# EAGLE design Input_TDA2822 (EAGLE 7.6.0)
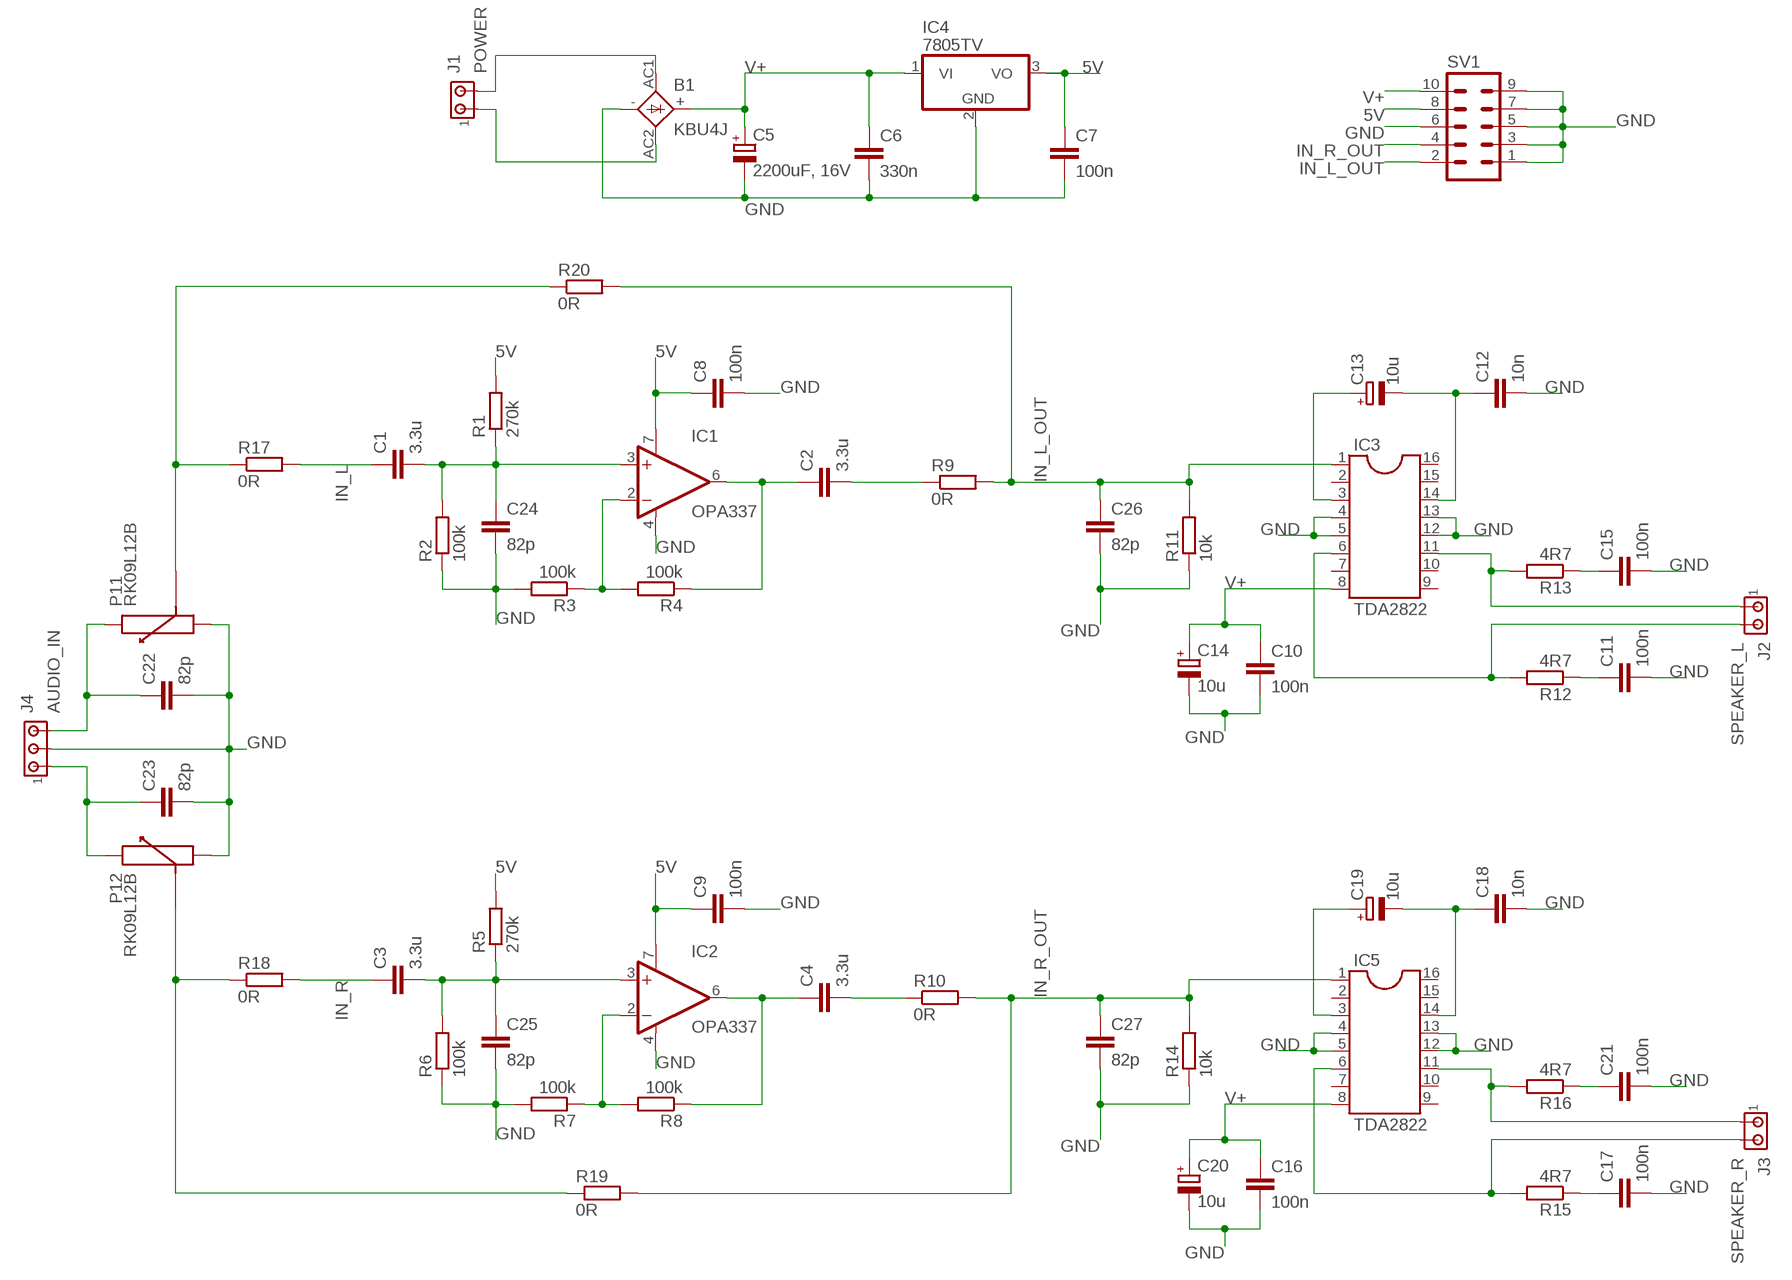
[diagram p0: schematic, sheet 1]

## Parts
B1  KBU4J  KBU  [KBU]
C1  3.3u  C-EU050-055X075  [C050-055X075]
C2  3.3u  C-EU050-055X075  [C050-055X075]
C3  3.3u  C-EU050-055X075  [C050-055X075]
C4  3.3u  C-EU050-055X075  [C050-055X075]
C5  2200uF, 16V  CPOL-EUE5-13  [E5-13]
C6  330n  C-EU050-035X075  [C050-035X075]
C7  100n  C-EU050-025X075  [C050-025X075]
C8  100n  C-EU050-025X075  [C050-025X075]
C9  100n  C-EU050-025X075  [C050-025X075]
C10  100n  C-EU050-025X075  [C050-025X075]
C11  100n  C-EU050-025X075  [C050-025X075]
C12  10n  C-EU025-025X050  [C025-025X050]
C13  10u  CPOL-EUE2-5  [E2-5]
C14  10u  CPOL-EUE2-5  [E2-5]
C15  100n  C-EU050-025X075  [C050-025X075]
C16  100n  C-EU050-025X075  [C050-025X075]
C17  100n  C-EU050-025X075  [C050-025X075]
C18  10n  C-EU025-025X050  [C025-025X050]
C19  10u  CPOL-EUE2-5  [E2-5]
C20  10u  CPOL-EUE2-5  [E2-5]
C21  100n  C-EU050-025X075  [C050-025X075]
C22  82p  C-EU025-024X044  [C025-024X044]
C23  82p  C-EU025-024X044  [C025-024X044]
C24  82p  C-EU025-024X044  [C025-024X044]
C25  82p  C-EU025-024X044  [C025-024X044]
C26  82p  C-EU025-024X044  [C025-024X044]
C27  82p  C-EU025-024X044  [C025-024X044]
IC1  OPA337  OPA336P  [DIL08]
IC2  OPA337  OPA336P  [DIL08]
IC3  TDA2822  DIL16S  [SOCKET-16]
IC4  7805TV  [TO220V]
IC5  TDA2822  DIL16S  [SOCKET-16]
J1  POWER  350428-1  [350428-1]
J2  SPEAKER_L  350428-1  [350428-1]
J3  SPEAKER_R  350428-1  [350428-1]
J4  AUDIO_IN  350429-1  [350429-1]
P1  RK09L12B  [ALPS-RK09L12B0]
R1  270k  R-EU_0309/V  [0309V]
R2  100k  R-EU_0309/V  [0309V]
R3  100k  R-EU_0309/V  [0309V]
R4  100k  R-EU_0309/V  [0309V]
R5  270k  R-EU_0309/V  [0309V]
R6  100k  R-EU_0309/V  [0309V]
R7  100k  R-EU_0309/V  [0309V]
R8  100k  R-EU_0309/V  [0309V]
R9  0R  R-EU_R0603  [R0603]
R10  0R  R-EU_R0603  [R0603]
R11  10k  R-EU_0309/V  [0309V]
R12  4R7  R-EU_0309/V  [0309V]
R13  4R7  R-EU_0309/V  [0309V]
R14  10k  R-EU_0309/V  [0309V]
R15  4R7  R-EU_0309/V  [0309V]
R16  4R7  R-EU_0309/V  [0309V]
R17  0R  R-EU_R0603  [R0603]
R18  0R  R-EU_R0603  [R0603]
R19  0R  R-EU_R0603  [R0603]
R20  0R  R-EU_R0603  [R0603]
SV1  ML10  [ML10]

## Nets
5V: C7.1 C8.1 C9.1 IC1.7(V+) IC2.7(V+) IC4.3(VO) R1.2 R5.2 SV1.8
GND: B1.- C5.- C6.2 C7.2 C8.2 C9.2 C10.2 C11.2 C12.2 C14.- C15.2 C16.2 C17.2 C18.2 C20.- C21.2 C22.2 C23.2 C24.2 C25.2 C26.2 C27.2 IC1.4(V-) IC2.4(V-) IC3.4 IC3.5 IC3.12 IC3.13 IC4.2(GND) IC5.4 IC5.5 IC5.12 IC5.13 J4.2 P1.GND1(1:GND$1) P1.GND2(2:GND$1) R2.1 R3.2 R6.1 R7.2 R11.1 R14.1 SV1.1 SV1.3 SV1.5 SV1.6 SV1.7 SV1.9
IN_L: C1.1 R17.2
IN_L_OUT: C26.1 IC3.1 R9.2 R11.2 R20.2 SV1.2
IN_R: C3.1 R18.2
IN_R_OUT: C27.1 IC5.1 R10.2 R14.2 R19.2 SV1.4
N$1: C1.2 C24.1 IC1.3(+IN) R1.1 R2.2
N$2: C3.2 C25.1 IC2.3(+IN) R5.1 R6.2
N$3: IC1.2(-IN) R3.1 R4.2
N$4: IC2.2(-IN) R7.1 R8.2
N$5: C2.1 IC1.6(OUT) R4.1
N$6: C4.1 IC2.6(OUT) R8.1
N$7: B1.AC1 J1.2
N$8: B1.AC2 J1.1
N$10: IC3.6 J2.2 R12.2
N$12: C2.2 R9.1
N$14: C19.+ IC5.3
N$15: C13.+ IC3.3
N$16: C12.1 C13.- IC3.14
N$17: C11.1 R12.1
N$18: C18.1 C19.- IC5.14
N$19: IC5.6 J3.2 R15.2
N$20: C17.1 R15.1
N$21: IC3.11 J2.1 R13.2
N$22: C15.1 R13.1
N$23: IC5.11 J3.1 R16.2
N$24: C21.1 R16.1
N$25: C22.1 J4.3 P1.IN1(1:IN$1)
N$27: C23.1 J4.1 P1.IN2(2:IN$1)
N$28: P1.OUT2(2:OUT$1) R18.1 R19.1
N$29: P1.OUT1(1:OUT$1) R17.1 R20.1
N$30: C4.2 R10.1
V+: B1.+ C5.+ C6.1 C10.1 C14.+ C16.1 C20.+ IC3.8 IC4.1(VI) IC5.8 SV1.10
Unconnected: IC3.2 IC3.7 IC3.9 IC3.10 IC3.15 IC3.16 IC5.2 IC5.7 IC5.9 IC5.10 IC5.15 IC5.16

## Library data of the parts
B1 = rectifier:KBU: DIOTEC RECTIFIER
C1-C4 C6-C12 C15-C18 C21-C27 = rcl:C-EU: CAPACITOR, European symbol
C5 C13 C14 C19 C20 = rcl:CPOL-EU: POLARIZED CAPACITOR, European symbol
IC1 IC2 = burr-brown:OPA336: CMOS Operational Amplifiers Single-Supply, MicroPower, MicroAmplifier(TM) Series; OC_FARNELL: unknown; OC_NEWARK: unknown
IC3 IC5 = ic-package:DIL16: Dual In Line / Socket
IC4 = linear:78*: Positive VOLTAGE REGULATOR Source: http://cache.national.com/ds/LM/LM78L05.pdf http://www.fairchildsemi.com/ds/LM/LM7805.pdf
J1-J3 = con-amp:350428-1: Universal MATE-N-LOK .250" Centerline, 600 V, 19 - 36 A max
J4 = con-amp:350429-1: Universal MATE-N-LOK .250" Centerline, 600 V, 19 - 36 A max Source: http://catalog.tycoelectronics.com/ .. ENG_CD_350429_Y.pdf
P1 = my:RK09L12B
R1-R20 = rcl:R-EU_: RESISTOR, European symbol
SV1 = con-ml:ML10: HARTING; OC_FARNELL: unknown; OC_NEWARK: unknown

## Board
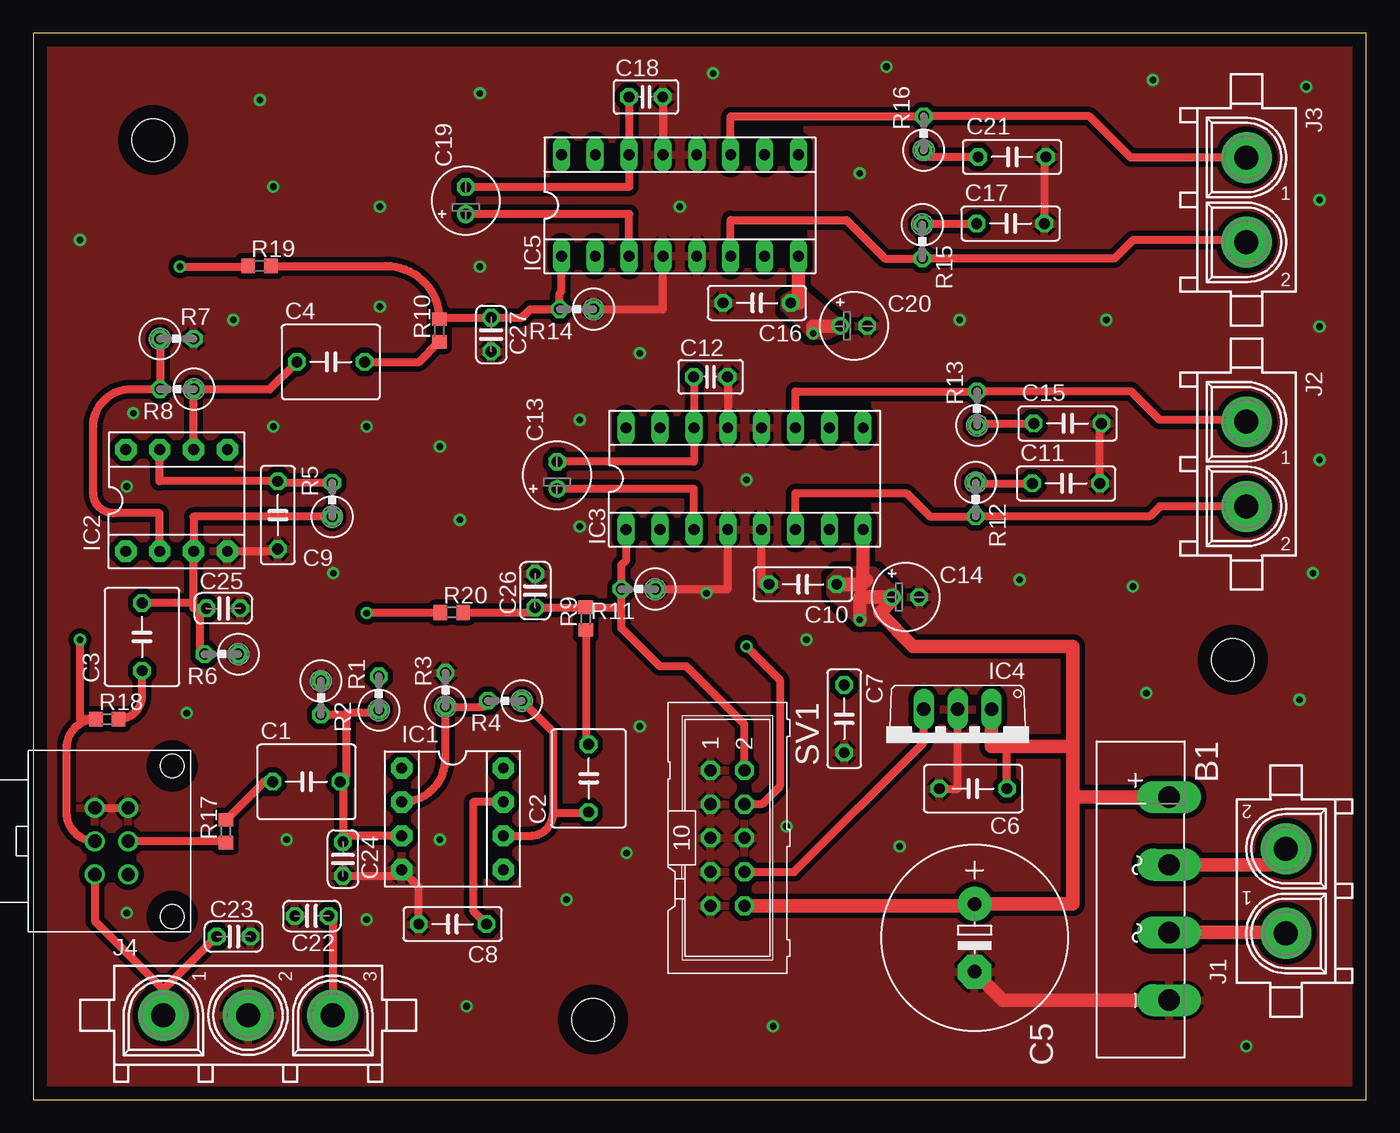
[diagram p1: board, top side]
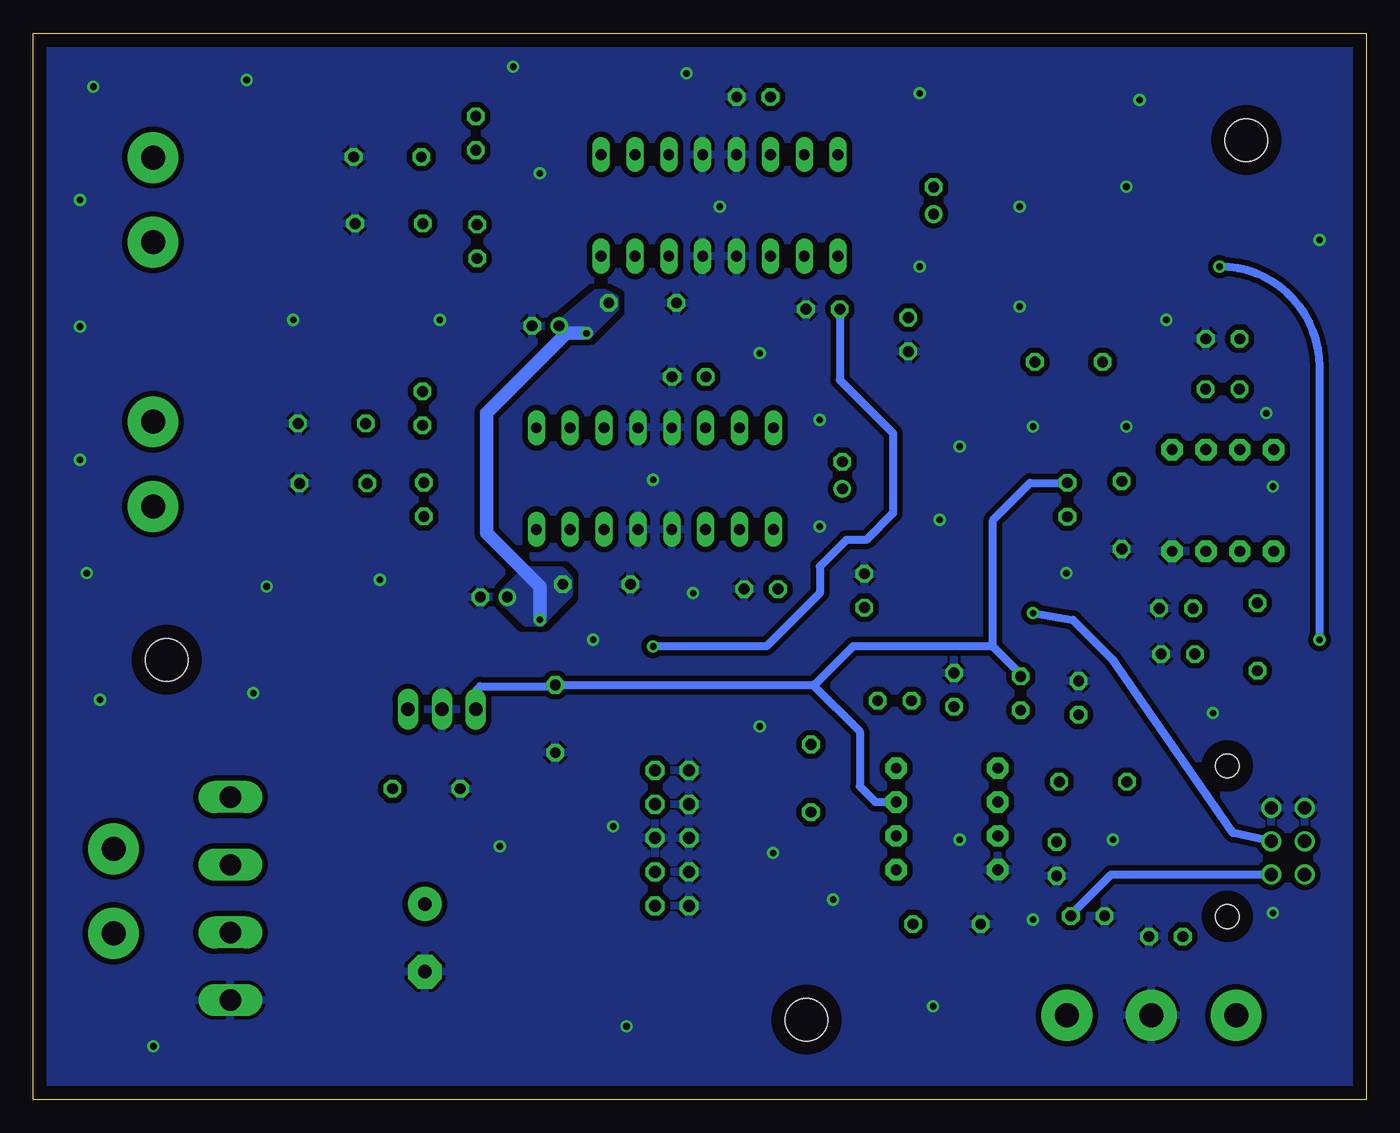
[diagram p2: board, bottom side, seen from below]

Size 100 x 80 mm. Coordinates in mm from the lower left corner, seen from the top.
Outline: 0,0 100,0 100,80 0,80 0,0
Copper layers (1*16): Top 0.035mm / dielectric 1.5mm / Bottom 0.035mm
Design rules "default": minimum track width 10mil, minimum drill 24mil, track to track 8mil, track to pad 8mil, pad to pad 8mil, via to via 8mil, smd to smd 8mil, copper to edge 40mil, drill to drill 8mil, minimum pad ring 10mil, minimum via ring 8mil, stop-mask expansion 4mil, vias tented up to drill 0mil, thermal gap 10mil
Holes 3.2 mm at 9,72 90,33 42,6

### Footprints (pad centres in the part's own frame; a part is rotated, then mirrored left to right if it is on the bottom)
KBU = drill 1.6 long: + -7.62,2.54; - 7.62,2.54; AC1 -2.54,2.54; AC2 2.54,2.54
C050-055X075 = drill 0.813 octagon: 1 -2.54,0; 2 2.54,0
E5-13 = drill 1.016 pad 2.54: + -2.54,0 | drill 1.016 pad 2.54 octagon: - 2.54,0
C050-035X075 = drill 0.813 octagon: 1 -2.54,0; 2 2.54,0
C050-025X075 = drill 0.813 octagon: 1 -2.54,0; 2 2.54,0
C025-025X050 = drill 0.813 octagon: 1 -1.27,0; 2 1.27,0
E2-5 = drill 0.813 pad 1.27: + -1.016,0 | drill 0.813 pad 1.27 octagon: - 1.016,0
C025-024X044 = drill 0.813 octagon: 1 -1.27,0; 2 1.27,0
DIL08 = drill 0.813 pad 1.6 octagon: 1 -3.81,-3.81; 2 -1.27,-3.81; 3 1.27,-3.81; 4 3.81,-3.81; 5 3.81,3.81; 6 1.27,3.81; 7 -1.27,3.81; 8 -3.81,3.81
SOCKET-16 = drill 0.813 long: 1 -8.89,-3.81; 2 -6.35,-3.81; 3 -3.81,-3.81; 4 -1.27,-3.81; 5 1.27,-3.81; 6 3.81,-3.81; 7 6.35,-3.81; 8 8.89,-3.81; 9 8.89,3.81; 10 6.35,3.81; 11 3.81,3.81; 12 1.27,3.81; 13 -1.27,3.81; 14 -3.81,3.81; 15 -6.35,3.81; 16 -8.89,3.81
TO220V = drill 1.016 long: 1 -2.54,-2.54; 2 0,-2.54; 3 2.54,-2.54
350428-1 = drill 1.8 pad 3.81: 1 -3.175,0; 2 3.175,0
350429-1 = drill 1.8 pad 3.81: 1 -6.35,0; 2 0,0; 3 6.35,0
ALPS-RK09L12B0 = drill 1: GND1 3.3,-2.5; GND2 5.8,-2.5; IN1 3.3,2.5; IN2 5.8,2.5; OUT1 3.3,0; OUT2 5.8,0 | hole 1.8: 0,-5.65; 0,5.65
0309V = drill 0.813 octagon: 1 -1.27,0; 2 1.27,0
R0603 = smd 1 x 1.1: 1 -0.85,0; 2 0.85,0
ML10 = drill 0.914 octagon: 1 -5.08,-1.27; 2 -5.08,1.27; 3 -2.54,-1.27; 4 -2.54,1.27; 5 0,-1.27; 6 0,1.27; 7 2.54,-1.27; 8 2.54,1.27; 9 5.08,-1.27; 10 5.08,1.27

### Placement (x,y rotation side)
B1  82.68,15.07 270 top
C1  20.49,23.84 0 top
C2  41.66,24.1 90 top
C3  8.16,34.71 90 top
C4  22.32,55.34 0 top
C5  70.62,12.13 270 top
C6  70.51,23.32 180 top
C7  60.84,28.57 270 top
C8  31.46,13.16 180 top
C9  18.34,43.85 270 top
C10  57.74,38.66 180 top
C11  77.49,46.23 0 top
C12  50.81,54.23 0 top
C13  39.3,46.84 90 top
C14  65.45,37.7 0 top
C15  77.6,50.73 0 top
C16  54.29,59.77 180 top
C17  73.32,65.73 0 top
C18  45.96,75.23 0 top
C19  32.45,67.45 90 top
C20  61.56,58.05 0 top
C21  73.43,70.73 0 top
C22  20.89,13.77 180 top
C23  15.03,12.23 0 top
C24  23.23,18.05 270 top
C25  14.26,36.85 0 top
C26  37.65,38.18 90 top
C27  34.35,57.4 270 top
IC1  31.45,21.05 270 top
IC2  10.75,44.95 0 top
IC3  53.37,46.59 0 top
IC4  69.35,26.74 180 top
IC5  48.51,67.09 0 top
J1  93.98,15.64 90 top
J2  91.02,47.68 270 top
J3  91.02,67.5 270 top
J4  16.11,6.32 0 top
P1  10.42,19.38 180 top
R1  25.92,30.48 90 top
R2  21.58,30.14 270 top
R3  30.92,30.74 90 top
R4  35.38,29.92 180 top
R5  22.42,45 90 top
R6  14.12,33.42 180 top
R7  10.76,57.08 0 top
R8  10.78,53.3 180 top
R9  41.45,36.08 90 top
R10  30.45,57.71 90 top
R11  45.4,38.3 180 top
R12  70.7,45.02 270 top
R13  70.8,51.86 90 top
R14  40.76,59.3 180 top
R15  66.7,64.38 270 top
R16  66.8,72.5 90 top
R17  14.45,20.13 90 top
R18  5.55,28.55 0 top
R19  16.97,62.55 0 top
R20  31.39,36.55 0 top
SV1  52.08,19.62 270 top

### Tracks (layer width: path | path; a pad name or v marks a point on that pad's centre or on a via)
5V
  Top 0.61: IC2.7 9.48,46.39 C9.1 18.34,46.27 R5.2 | IC1.7 33,22.32 33,14.16 C8.1 | SV1.8 57.08,17.08 66.81,26.81 IC4.3
  Bottom 0.61: IC4.3 66.81,30.69 66.5,31 60.45,31 C7.1 41.5,31.11 | 41.5,31.11 41.39,31.11 38.5,34 28,34 | IC1.7 36.82,22.32 38,23.5 38,27.61 41.5,31.11 | 28,34 28,43.5 25.23,46.27 R5.2 | R1.2 26.25,32.25 28,34
GND  (via drill 0.5)
  Top 0.61: J4.2 16.3,6.51 | P1.GND2 P1.GND1 | IC2.4 18.34,41.14 C9.2 | C24.2 27.18,16.78 IC1.4 28.92,15.96 C8.2 | C10.2 54.64,38.66 IC3.5 | C11.2 80.03,50.73 C15.2 | C18.2 IC5.13 | C12.2 52.1,54.23 IC3.13 | R11.1 52.1,38.3 IC3.4 | R14.1 47.24,59.3 IC5.4 | C21.2 75.86,70.62 C17.2 | C6.2 69.35,23.32 IC4.2
  Top 1.016: B1.- 72.76,7.45 C5.-
  other vias: 17,75 30.5,49 45.5,56 48.5,67 51,77 62,69.5 84,76.5 80.5,58.5 69.5,58.5 82.5,38.5 74,39 83.5,30.5 50.5,38 45.5,28 40,15 22.5,39.5 11.5,29 3.5,64.5 7,46 18,50.5 26,59.5 26,67 7.5,51.5 33.5,62.5 41,51 32,43.5 41,43 44.5,18.5 30.5,19.5 25,13.5 19,19.5 7,14 32.5,7 55.5,5.5 91,4 95,30 65,19 58,34.5 56.5,20.5 64,77.5 96.5,58 95.5,76 96,39.5 96.5,48 96.5,67.5 33.5,75.5 18,68.5 25,50.5 15,58.5 53.5,46.5
  pour Top (isolate 0.406, rank 2): 0.5,79.5 0.5,0.5 99.5,0.5 99.5,79.5
  pour Bottom (isolate 0.406, rank 2): 0.5,79.5 0.5,0.5 99.5,0.5 99.5,79.5
IN_L
  Top 0.61: R17.2 17.31,23.84 C1.1
IN_L_OUT
  Top 0.61: R11.2 44.13,40.13 44.5,40.5 44.5,42.76 IC3.1 | R20.2 37.29,36.55 C26.1 41.43,36.91 R9.2 44.13,36.93 R11.2 | SV1.2 53.35,28.15 49,32.5 47,32.5 44.13,35.37 R11.2
IN_R
  Top 0.61: R18.2 arc90 8.16,30.31 C3.1
IN_R_OUT  (via drill 0.5)
  Top 0.61: IC5.1 39.62,60.62 39.49,60.49 R14.2 37.3,59.3 36.67,58.67 C27.1 30.56,58.67 R10.2 arc90 26.46,62.55 R19.2 | SV1.4 54.66,22.16 56,23.5 56,31.5 v53.5,34
  Bottom 0.61: R14.2 39.49,53.99 35.5,50 35.5,44 37.5,42 39,42 41,40 41,38 45,34 v53.5,34
N$1
  Top 0.61: IC1.3 23.69,19.78 C24.1 23.23,23.64 C1.2 23.5,24.31 23.5,29 | 23.5,29 23.37,28.87 R2.2 | R1.1 25.71,29 23.5,29
N$2
  Top 0.61: IC2.3 arc90 12,41.12 12,39 | 12.02,37.25 C3.2 | 12.02,37.25 IC2.3 | C25.1 12.5,36.85 | 12.5,36.85 12.02,36.85 12.02,37.25 | R6.2 12.5,33.42 12.5,36.85 | R5.1 12.02,43.73 IC2.3
N$3
  Top 0.61: IC1.2 arc90 30.92,25.6 R3.1 33.66,29.47 arc90 R4.2
N$4
  Top 0.61: IC2.2 9.48,44 6,44 arc-90 4.5,45.5 4.5,50.5 arc-90 7.3,53.3 R8.2 9.51,57.06 arc90 R7.1
N$5
  Top 0.61: IC1.6 37.28,19.78 arc90 39,21.5 | 39,21.5 41.6,21.5 arc90 C2.1 | R4.1 39,27.57 39,21.5
N$6
  Top 0.61: C4.1 17.74,53.3 R8.1 12.02,53.27 IC2.6
N$7
  Top 1.016: J1.2 92.78,17.61 B1.AC1
N$8
  Top 1.016: J1.1 93.92,12.53 B1.AC2
N$10
  Top 0.61: IC3.6 57.18,45.5 65.5,45.5 67.25,43.75 R12.2 83.75,43.75 84.5,44.5 J2.2
N$12
  Top 0.61: R9.1 41.45,26.85 C2.2
N$14
  Top 0.61: IC5.3 44.7,66.43 C19.+
N$15
  Top 0.61: IC3.3 49.56,45.82 C13.+
N$16
  Top 0.61: C12.1 49.56,54.23 IC3.14 49.56,47.86 C13.-
N$17
  Top 0.61: R12.1 70.7,46.23 C11.1
N$18
  Top 0.61: C18.1 IC5.14 44.7,68.47 C19.-
N$19
  Top 0.61: J3.2 90.84,64.5 82.5,64.5 81.11,63.11 R15.2 63.89,63.11 61,66 52.32,66 IC5.6
N$20
  Top 0.61: R15.1 66.78,65.73 C17.1
N$21
  Top 0.61: J2.1 90.88,51 84.5,51 82.37,53.13 R13.2 57.18,53.13 IC3.11
N$22
  Top 0.61: R13.1 70.8,50.73 C15.1
N$23
  Top 0.61: IC5.11 52.32,73.77 R16.2 79.23,73.77 82.33,70.67 J3.1
N$24
  Top 0.61: R16.1 67.3,70.73 C21.1
N$25
  Top 0.61: J4.3 22.5,6.36 22.5,13.43 C22.1
  Bottom 0.61: C22.1 22.16,13.84 19.12,16.88 P1.IN1
N$27
  Top 0.61: 9.76,8.26 J4.1 | P1.IN2 4.62,13.4 9.76,8.26 | 9.76,8.26 9.79,8.26 C23.1
N$28  (via drill 0.5)
  Top 0.61: P1.OUT2 arc-90 2.5,21.5 2.5,26.35 arc-90 R18.1 3.5,28.55 v3.5,34.5 | v11,62.5 16.07,62.5 arc90 R19.1
  Bottom 0.61: v3.5,34.5 3.5,55 arc-90 v11,62.5
N$29  (via drill 0.5)
  Top 0.61: R20.1 30.49,36.5 v25,36.5 | R17.1 14.35,19.38 P1.OUT1
  Bottom 0.61: v25,36.5 22,36 19,33 10,20 P1.OUT1
N$30
  Top 0.61: C4.2 28.93,55.34 R10.1
V+  (via drill 0.5)
  Top 0.61: C6.1 73.05,26.5 74.5,26.5
  Top 1.016: B1.+ 78,22.69 | 78,22.69 78,26.5 | 78,26.5 74.5,26.5 71.89,26.5 IC4.1 | 78,22.69 78,14.67 C5.+ 70.62,14.54 SV1.10 | C20.+ 58.5,58.05 v58.5,57.5 | v62,36 62,37.7 C14.+ 64.43,37.43 63.5,36.5 66,34 78,34 78,26.5 | IC3.8 62.26,39.24 62.5,39 62.16,38.66 C10.1 | IC5.8 57.4,59.77 C16.1
  Bottom 1.016: v62,36 62,38.5 66,42.5 66,51.5 60,57.5 v58.5,57.5
  pour Top (isolate 0.406, no thermals): 58.5,57.5 56.5,59.5 56.5,60 57.5,60.5 60.5,58 59.5,57.5
  pour Bottom (isolate 0.406, no thermals): 58.5,57.5 56.5,59.5 56.5,60 57.5,60.5 60.5,58 59.5,57.5
  pour Bottom (isolate 0.406, no thermals): 62,36 60,38 60,38.5 60,39 60.5,39.5 63,39.5 64.5,38 64.5,37.5 63,36
  pour Top (isolate 0.406, no thermals): 62,36 60,38 60,38.5 60,39 60.5,39.5 63,39.5 64.5,38 64.5,37.5 63,36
